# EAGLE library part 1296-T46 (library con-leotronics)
1.27mm SINGLE ROW FEMALE SOCKET Source: http://www.leotronics.co.uk/Conexcon/Data%20Sheets/sec.%20A/1296ing.pdf
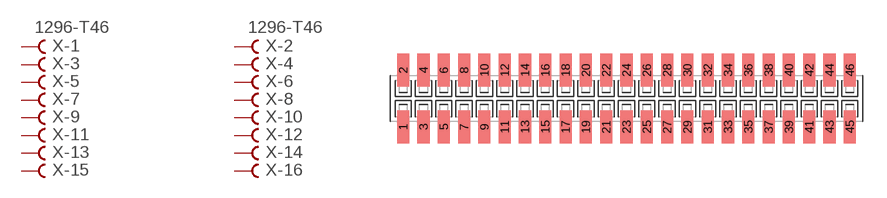
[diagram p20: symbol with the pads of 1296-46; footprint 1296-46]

Designator prefix X; gates -1=FVAL -2=FVAL -3=F -4=F -5=F -6=F -7=F -8=F -9=F -10=F -11=F -12=F -13=F -14=F -15=F -16=F -17=F -18=F -19=F -20=F -21=F -22=F -23=F -24=F -25=F -26=F -27=F -28=F -29=F -30=F -31=F -32=F -33=F -34=F -35=F -36=F -37=F -38=F -39=F -40=F -41=F -42=F -43=F -44=F -45=F -46=F

## 1296-T46 (OC_FARNELL: unknown; OC_NEWARK: unknown)  [1296-46]
1  -1:B  pas
2  -2:B  pas
3  -3:B  pas
4  -4:B  pas
5  -5:B  pas
6  -6:B  pas
7  -7:B  pas
8  -8:B  pas
9  -9:B  pas
10  -10:B  pas
11  -11:B  pas
12  -12:B  pas
13  -13:B  pas
14  -14:B  pas
15  -15:B  pas
16  -16:B  pas
17  -17:B  pas
18  -18:B  pas
19  -19:B  pas
20  -20:B  pas
21  -21:B  pas
22  -22:B  pas
23  -23:B  pas
24  -24:B  pas
25  -25:B  pas
26  -26:B  pas
27  -27:B  pas
28  -28:B  pas
29  -29:B  pas
30  -30:B  pas
31  -31:B  pas
32  -32:B  pas
33  -33:B  pas
34  -34:B  pas
35  -35:B  pas
36  -36:B  pas
37  -37:B  pas
38  -38:B  pas
39  -39:B  pas
40  -40:B  pas
41  -41:B  pas
42  -42:B  pas
43  -43:B  pas
44  -44:B  pas
45  -45:B  pas
46  -46:B  pas

## Footprint 1296-46 (pad centres in mm)
1.27mm SINGLE ROW FEMALE SOCKET Source: http://www.leotronics.co.uk/Conexcon/Data%20Sheets/sec.%20A/1296ing.pdf
smd 0.76 x 2.05: 1 -13.97,-1.78; 2 -13.97,1.78; 3 -12.7,-1.78; 4 -12.7,1.78; 5 -11.43,-1.78; 6 -11.43,1.78; 7 -10.16,-1.78; 8 -10.16,1.78; 9 -8.89,-1.78; 10 -8.89,1.78; 11 -7.62,-1.78; 12 -7.62,1.78; 13 -6.35,-1.78; 14 -6.35,1.78; 15 -5.08,-1.78; 16 -5.08,1.78; 17 -3.81,-1.78; 18 -3.81,1.78; 19 -2.54,-1.78; 20 -2.54,1.78; 21 -1.27,-1.78; 22 -1.27,1.78; 23 0,-1.78; 24 0,1.78; 25 1.27,-1.78; 26 1.27,1.78; 27 2.54,-1.78; 28 2.54,1.78; 29 3.81,-1.78; 30 3.81,1.78; 31 5.08,-1.78; 32 5.08,1.78; 33 6.35,-1.78; 34 6.35,1.78; 35 7.62,-1.78; 36 7.62,1.78; 37 8.89,-1.78; 38 8.89,1.78; 39 10.16,-1.78; 40 10.16,1.78; 41 11.43,-1.78; 42 11.43,1.78; 43 12.7,-1.78; 44 12.7,1.78; 45 13.97,-1.78; 46 13.97,1.78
